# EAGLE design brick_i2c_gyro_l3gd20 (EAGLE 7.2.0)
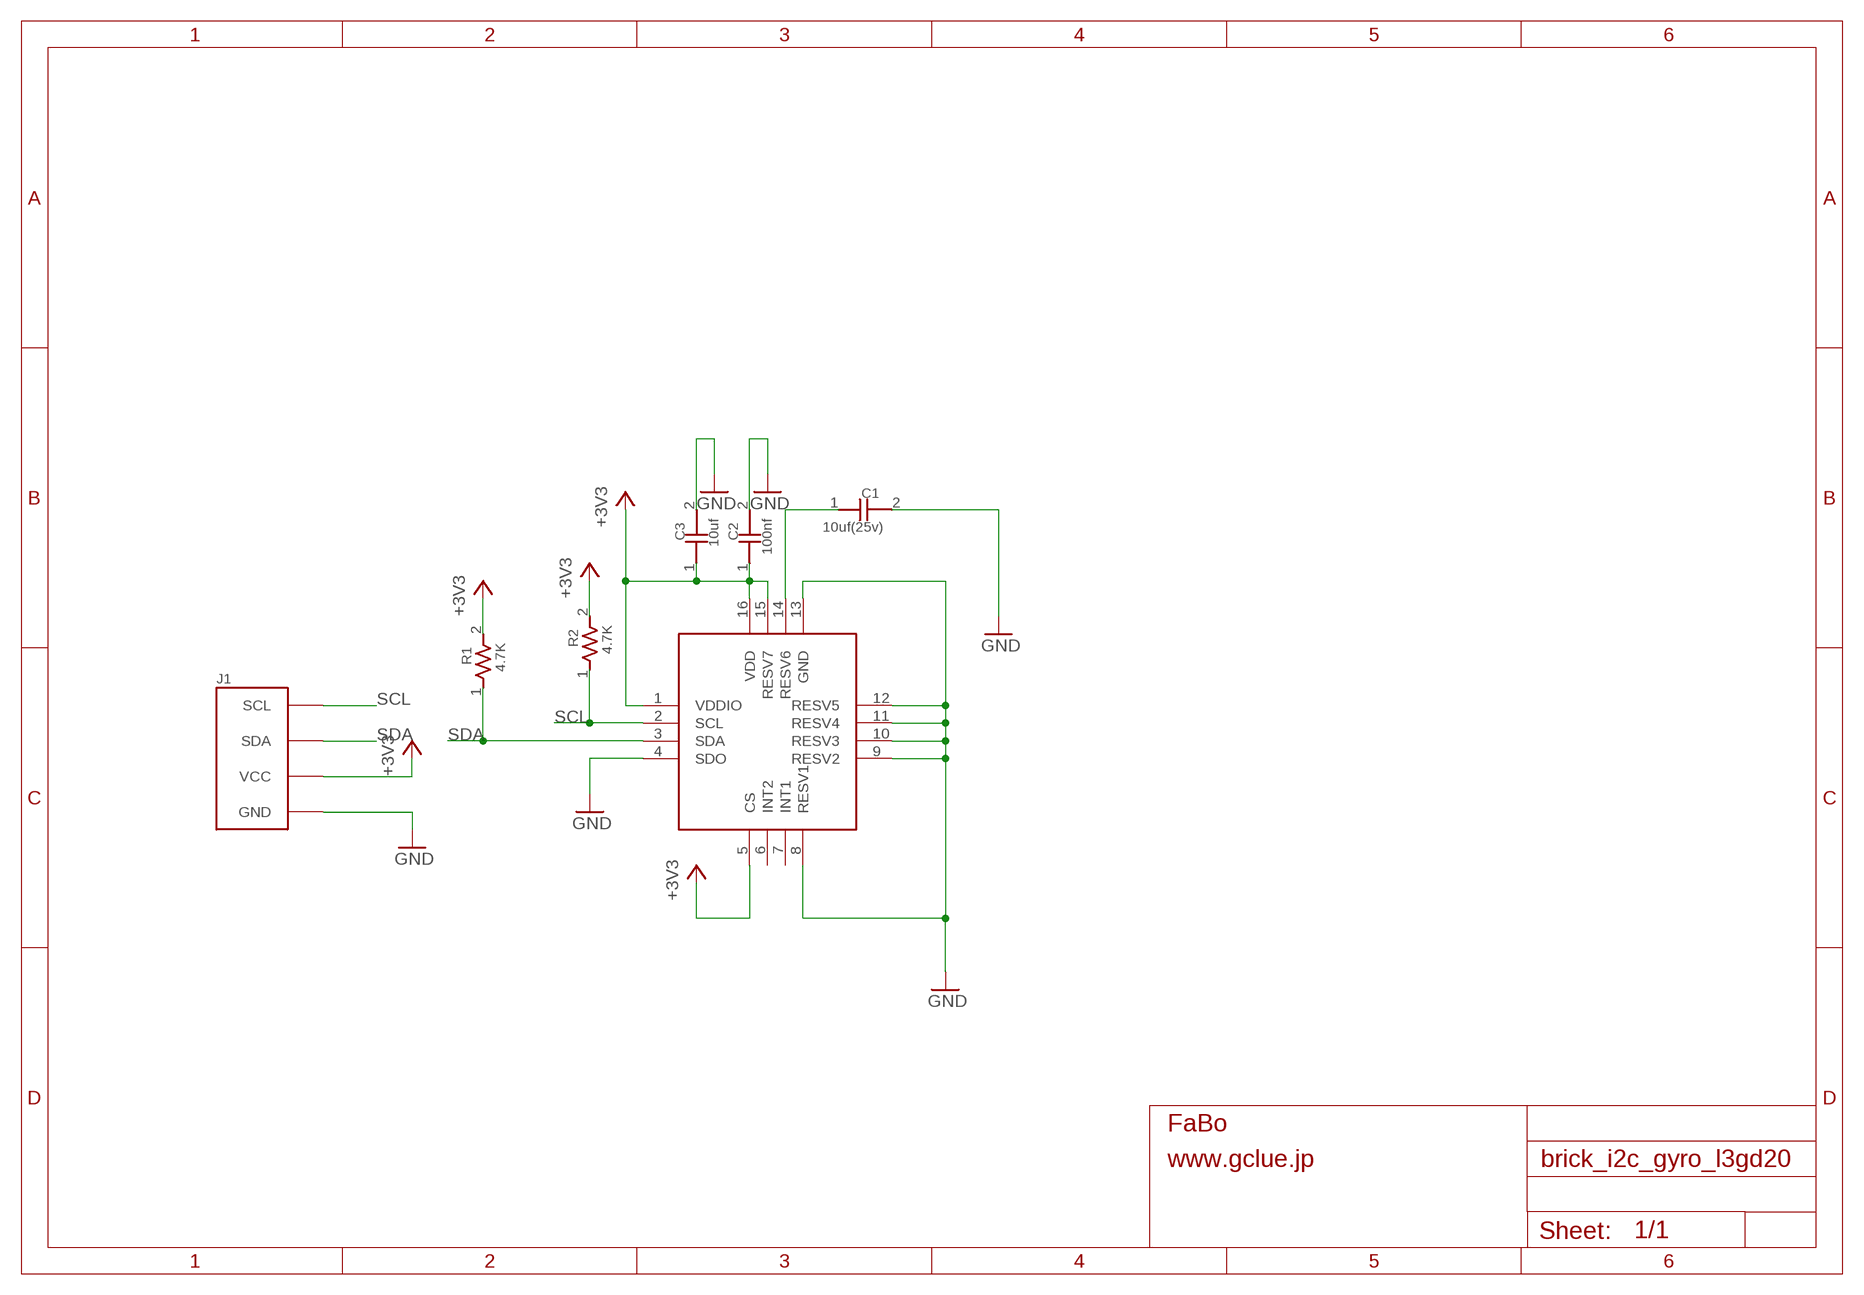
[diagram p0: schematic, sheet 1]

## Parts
C1  10uf(25v)  CAPACITOR0603  [0603]
C2  100nf  CAPACITOR0603  [0603]
C3  10uf  CAPACITOR0603  [0603]
J1  BRICK_I2C  [BRICK_I2C]
R1  4.7K  RESISTOR0603  [0603]
R2  4.7K  RESISTOR0603  [0603]
U$3  ST-L3GD20  [LGA-16]

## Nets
+3V3: C2.1 C3.1 J1.VCC R1.2 R2.2 U$3.1(VDDIO) U$3.5(CS) U$3.15(RESV7) U$3.16(VDD)
GND: C1.2 C2.2 C3.2 J1.GND U$3.4(SDO) U$3.8(RESV1) U$3.9(RESV2) U$3.10(RESV3) U$3.11(RESV4) U$3.12(RESV5) U$3.13(GND)
N$3: C1.1 U$3.14(RESV6)
SCL: J1.SCL R2.1 U$3.2(SCL)
SDA: J1.SDA R1.1 U$3.3(SDA)
Unconnected: U$3.6(INT2) U$3.7(INT1)

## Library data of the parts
C1-C3 = GClue-Capacitor:CAPACITOR
J1 = gclue:BRICK_I2C: FaBo Brick 4pin(I2C)
R1 R2 = GClue-Resistors:RESISTOR
U$3 = GClue-Mems:ST-L3GD20

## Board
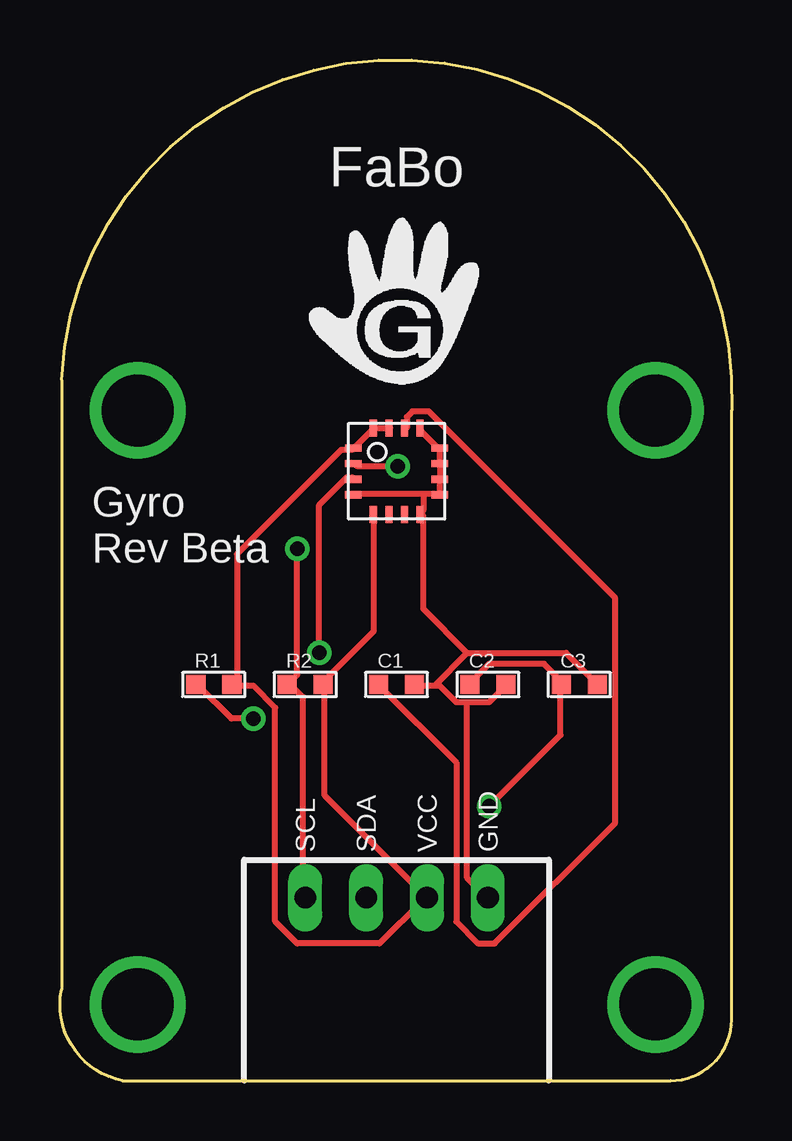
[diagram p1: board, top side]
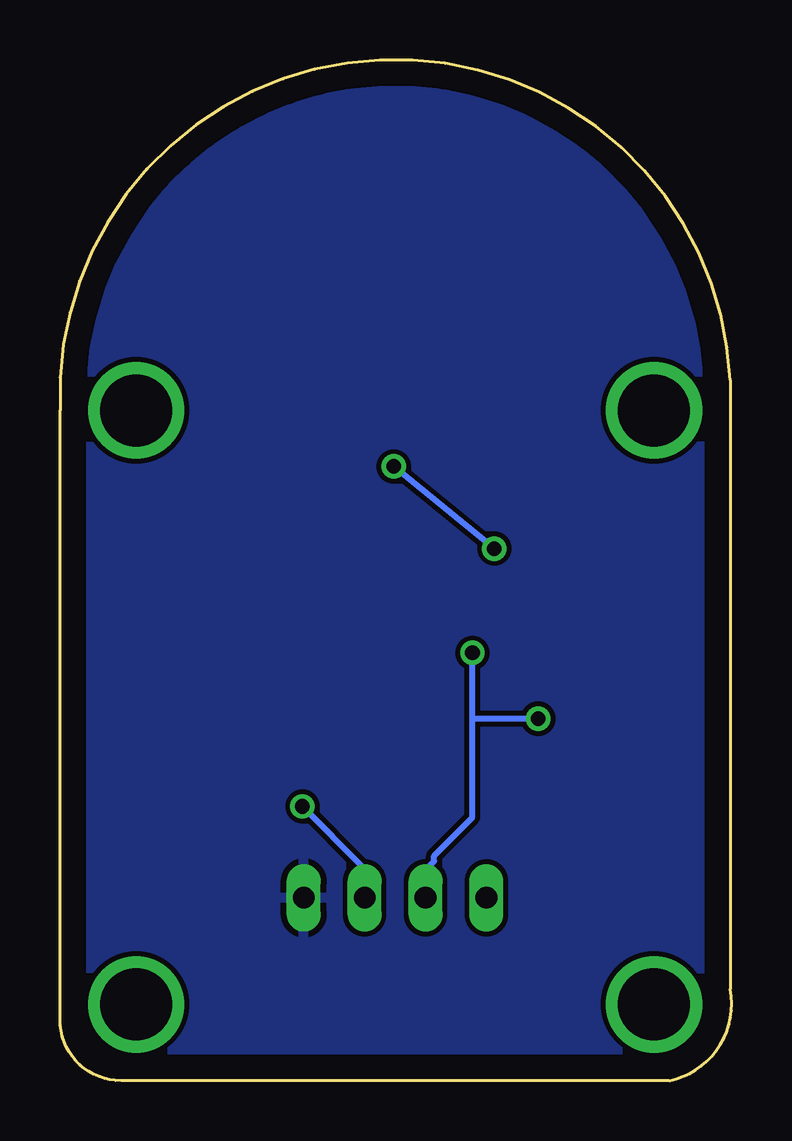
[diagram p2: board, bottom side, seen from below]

Size 28 x 42.55 mm. Coordinates in mm from the lower left corner, seen from the top.
Copper layers (1*16): Top 0.035mm / dielectric 1.5mm / Bottom 0.035mm
Design rules "default": minimum track width 10mil, minimum drill 24mil, track to track 8mil, track to pad 8mil, pad to pad 8mil, via to via 8mil, smd to smd 8mil, copper to edge 40mil, drill to drill 8mil, minimum pad ring 10mil, minimum via ring 8mil, stop-mask expansion 4mil, vias tented up to drill 0mil, thermal gap 10mil

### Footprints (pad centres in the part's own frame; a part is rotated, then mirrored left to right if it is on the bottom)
0603 = smd 0.8 x 0.8: 1 -0.75,0; 2 0.75,0
BRICK_I2C = drill 0.9 long: GND 3.81,-12.7; SCL -3.81,-12.7; SDA -1.27,-12.7; VCC 1.27,-12.7 | drill 3 pad 3.81: P$5 -10.795,7.62; P$6 10.795,7.62; P$7 -10.795,-17.145; P$8 10.795,-17.145
LGA-16 = smd 0.7 x 0.3: 1 -1.8,0.97; 2 -1.8,0.32; 3 -1.8,-0.33; 4 -1.8,-0.98; 9 1.8,-0.98; 10 1.8,-0.33; 11 1.8,0.32; 12 1.8,0.97 | smd 0.3 x 0.7: 5 -0.97,-1.8; 6 -0.32,-1.8; 7 0.33,-1.8; 8 0.98,-1.8; 13 0.98,1.8; 14 0.33,1.8; 15 -0.32,1.8; 16 -0.97,1.8

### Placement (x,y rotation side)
C1  14.03,16.51 0 top
C2  17.84,16.51 0 top
C3  21.65,16.51 0 top
J1  14.03,20.32 0 top
R1  6.41,16.51 0 top
R2  10.22,16.51 0 top
U$3  14.03,25.4 0 top

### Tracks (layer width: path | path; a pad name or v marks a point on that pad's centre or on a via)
+3V3  (via drill 0.61)
  Top 0.254: 13.09,27.2 12.41,26.52 U$3.1 12.18,26.29 11.72,26.29 7.38,21.95 7.38,16.69 R1.2 7.38,16.46 8.06,16.46 8.98,15.54 8.98,6.63 9.89,5.71 13.32,5.71 15.15,7.54 J1.VCC 11.04,11.89 11.04,16.46 R2.2 11.04,16.69 13.09,18.75 13.09,23.55 U$3.5 | 13.09,27.2 13.78,27.2 U$3.15 | 13.09,27.2 U$3.16 | C2.1 17.21,16.69 17.89,17.37 20.18,17.37 20.87,16.69 C3.1 20.87,16.46 20.87,14.4 v17.89,11.43
  Bottom 0.254: v17.89,11.43 15.38,8.91 15.38,7.77 J1.VCC
GND
  Top 0.254: 15.84,25.15 15.84,25.6 U$3.11 15.84,25.83 15.84,26.29 U$3.12 15.61,26.52 15.15,26.98 U$3.13 | 15.15,24.46 15.61,24.46 U$3.9 15.84,24.46 15.84,25.15 | 15.15,24.46 12.41,24.46 U$3.4 | 15.15,24.46 15.15,23.77 U$3.8 15.15,23.55 15.15,19.66 16.98,17.83 | 15.84,25.15 U$3.10 | 15.61,16.46 15.84,16.46 16.52,15.77 16.98,15.77 | 15.61,16.46 14.92,16.46 C1.2 | 16.98,15.77 17.89,15.77 18.58,16.46 C2.2 | 16.98,17.83 21.09,17.83 22.24,16.69 C3.2 | 15.61,16.46 16.98,17.83 | 16.98,15.77 16.98,8.46 17.66,7.77 J1.GND
  pour Bottom: 0.06,0 30.54,0 30.54,43.18 0.06,43.18
N$3
  Top 0.254: U$3.14 14.46,27.2 14.46,27.66 14.69,27.89 15.38,27.89 23.15,20.12 23.15,10.74 18.12,5.71 17.44,5.71 16.52,6.63 16.52,13.26 13.32,16.46 C1.1
SCL  (via drill 0.61)
  Top 0.254: v14.08,25.6 12.41,25.6 U$3.2 | v9.89,22.17 9.89,16.92 9.66,16.69 R2.1 9.66,16.46 10.12,16 10.12,7.77 J1.SCL
  Bottom 0.254: v9.89,22.17 v14.08,25.6
SDA  (via drill 0.61)
  Top 0.254: v10.81,17.83 10.81,24 11.95,25.15 12.18,25.15 U$3.3 | v8.06,15.09 7.15,15.09 5.78,16.46 R1.1
  Bottom 0.254: 10.81,15.09 10.81,10.97 12.41,9.37 12.41,9.14 12.64,8.91 12.64,7.77 J1.SDA | 10.81,15.09 v10.81,17.83 | 10.81,15.09 v8.06,15.09

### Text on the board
tPlace: Gyro / Rev Beta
